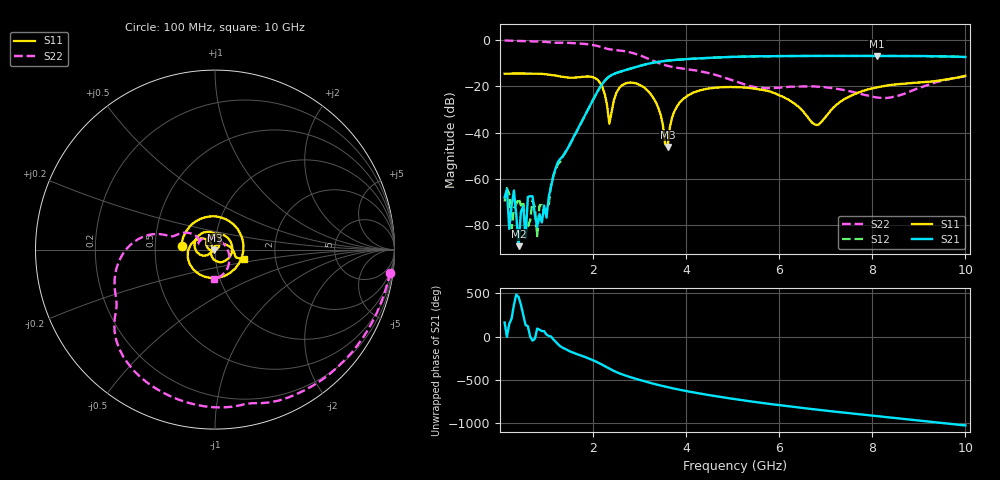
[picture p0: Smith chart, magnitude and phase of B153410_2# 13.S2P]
!  2-Port S-parameters saved by WinCal
! VAR MeasName=S-Parameters (CALIBRATED_DATA) read from VNA (N5245A)
! VAR MeasDate=2016-12-23 10:00:00
! VAR NAME=B153410_2# 13
! VAR FILENAME=B153410_2# 13.S2P
! VAR DATE=2016-12-23 10:00:00
! VAR PHYS_PORTS=1,2
# Hz S DB R 50
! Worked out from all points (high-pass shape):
!   199 points, 100 MHz to 10 GHz, reference 50 ohm
!   highest |S21| = -6.79 dB at 8.1 GHz (marker M1); lowest = -89.1 dB at 400 MHz (marker M2)
!   |S21| within 3 dB of the highest: 3.282 GHz to end of sweep
!   lowest |S11| = -46.2 dB at 3.6 GHz (marker M3), VSWR 1.01, Z = 49.7 - j0.363 ohm
!   |S11| at or under -10 dB: start of sweep to end of sweep
!   |S22| runs from -25.0 to -0.1 dB; largest |S21 - S12| = 0.0037
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1e8  -14.53 173.2  -67.99 163.3  -69.79 -133.9  -0.13 -7.4
1.5e8  -14.52 169.3  -64.45 -3.3  -64.00 -101.7  -0.18 -11.0
2e8  -14.50 165.9  -81.61 148.3  -66.45 157.4  -0.22 -14.3
2.5e8  -14.45 161.8  -71.65 -152.8  -81.48 56.9  -0.25 -17.6
3e8  -14.41 157.9  -64.99 7.9  -72.73 38.2  -0.28 -21.0
4e8  -14.42 149.8  -89.09 99.2  -68.42 -19.5  -0.33 -27.6
5.5e8  -14.40 136.2  -85.63 134.1  -79.89 -42.4  -0.41 -37.5
6.5e8  -14.41 126.3  -67.47 -2.7  -77.87 -2.6  -0.49 -44.1
7e8  -14.43 121.1  -67.55 -47.4  -69.38 1.2  -0.52 -47.4
8e8  -14.50 109.2  -80.67 92.3  -84.78 -83.6  -0.59 -53.9
1.75e9  -15.92 -98.0  -35.57 138.5  -35.48 138.2  -1.52 -113.5
2.15e9  -18.39 153.6  -20.38 46.6  -20.38 46.7  -2.82 -140.7
2.35e9  -36.10 153.5  -15.71 -12.7  -15.70 -12.6  -3.93 -149.6
2.7e9  -18.67 168.7  -12.93 -92.7  -12.92 -92.6  -4.86 -166.4
3.4e9  -29.15 45.5  -9.39 159.2  -9.38 159.3  -9.82 164.5
3.6e9  -46.18 -131.9  -8.86 133.4  -8.85 133.4  -11.09 163.5
3.95e9  -25.24 151.6  -8.30 93.5  -8.28 93.6  -12.34 161.7
5.05e9  -20.27 12.1  -7.19 -5.9  -7.20 -5.7  -17.75 144.5
6.7e9  -35.55 -178.6  -6.82 -120.7  -6.82 -120.7  -20.01 154.2
8.1e9  -20.40 1.6  -6.79 156.7  -6.81 156.7  -24.81 70.6
8.35e9  -19.50 -6.8  -6.83 142.4  -6.81 142.6  -24.91 39.4
1e10  -15.42 -18.8  -7.29 49.1  -7.31 49.4  -15.68 -91.1
